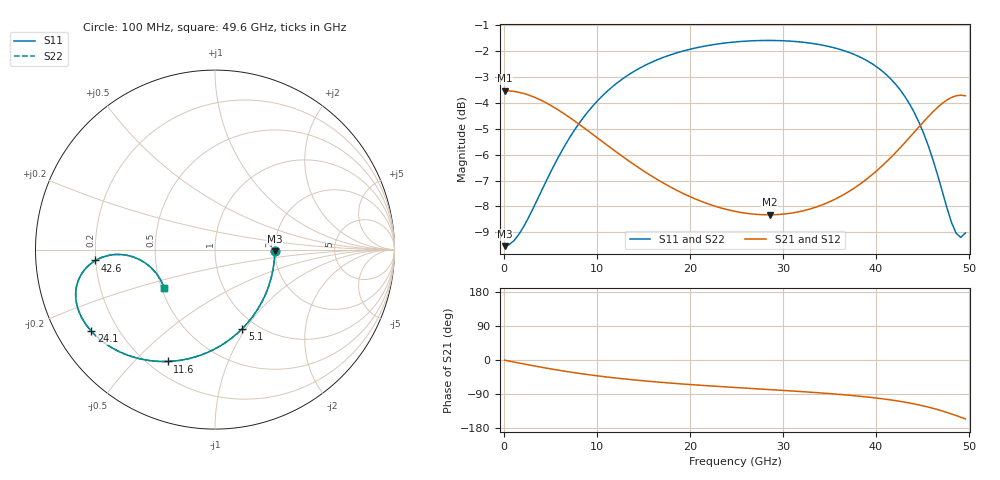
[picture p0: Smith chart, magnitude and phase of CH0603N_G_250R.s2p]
# GHz S RI R 250
! S-Parameters data
! Freq  reS11  imS11  reS21  imS21  reS12  imS12  reS22  imS22
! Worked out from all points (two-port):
!   100 points, 100 MHz to 49.6 GHz, reference 250 ohm
!   highest |S21| = -3.52 dB at 100 MHz (marker M1); lowest = -8.3 dB at 28.6 GHz (marker M2)
!   |S21| within 3 dB of the highest: start of sweep to 14.58 GHz; 40.38 GHz to end of sweep
!   lowest |S11| = -9.5 dB at 100 MHz (marker M3), VSWR 2.00, Z = 500 - j11.3 ohm
!   |S11| at or under -10 dB: nowhere
!   |S22| runs from -9.5 to -1.6 dB; largest |S21 - S12| = 0
!   S11 on the Smith chart (normalised r, x): 100 MHz: 2.00, -0.05; 5.1 GHz: 0.86, -0.97; 11.6 GHz: 0.27, -0.63; 24.1 GHz: 0.10, -0.30; 42.6 GHz: 0.20, -0.04; 49.6 GHz: 0.52, -0.25
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0.1  0.3333 -0.0101  0.6666 -0.00565  0.6666 -0.00565  0.3333 -0.0101
1.1  0.3236 -0.1098  0.6615 -0.0618  0.6615 -0.0618  0.3236 -0.1098
2.6  0.281 -0.2507  0.639 -0.1413  0.639 -0.1413  0.281 -0.2507
5.1  0.1522 -0.4404  0.5713 -0.2499  0.5713 -0.2499  0.1522 -0.4404
6.6  0.0556 -0.52  0.5208 -0.2972  0.5208 -0.2972  0.0556 -0.52
8.6  -0.078 -0.5874  0.4514 -0.3403  0.4514 -0.3403  -0.078 -0.5874
11.6  -0.2629 -0.6232  0.3558 -0.3724  0.3558 -0.3724  -0.2629 -0.6232
14.1  -0.3912 -0.6141  0.2895 -0.3808  0.2895 -0.3808  -0.3912 -0.6141
16.6  -0.4946 -0.5851  0.2354 -0.3807  0.2354 -0.3807  -0.4946 -0.5851
20.1  -0.6036 -0.5284  0.1764 -0.3757  0.1764 -0.3757  -0.6036 -0.5284
24.1  -0.6889 -0.4546  0.1254 -0.3715  0.1254 -0.3715  -0.6889 -0.4546
25.1  -0.7051 -0.4356  0.1144 -0.3713  0.1144 -0.3713  -0.7051 -0.4356
28.6  -0.748 -0.3679  0.0788 -0.3752  0.0788 -0.3752  -0.748 -0.3679
33.1  -0.7748 -0.2771  0.0326 -0.3931  0.0326 -0.3931  -0.7748 -0.2771
38.1  -0.7591 -0.1658  -0.04 -0.4354  -0.04 -0.4354  -0.7591 -0.1658
41.6  -0.6969 -0.0824  -0.1318 -0.4773  -0.1318 -0.4773  -0.6969 -0.0824
42.6  -0.6658 -0.0605  -0.1702 -0.4882  -0.1702 -0.4882  -0.6658 -0.0605
45.1  -0.5513 -0.0271  -0.3011 -0.4959  -0.3011 -0.4959  -0.5513 -0.0271
46.6  -0.457 -0.0404  -0.4041 -0.4681  -0.4041 -0.4681  -0.457 -0.0404
47.6  -0.3896 -0.0737  -0.4769 -0.4255  -0.4769 -0.4255  -0.3896 -0.0737
48.6  -0.328 -0.1312  -0.5436 -0.3591  -0.5436 -0.3591  -0.328 -0.1312
49.6  -0.2835 -0.2113  -0.5929 -0.2704  -0.5929 -0.2704  -0.2835 -0.2113
